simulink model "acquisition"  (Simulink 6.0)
settings: Solver=FixedStepDiscrete  StartTime=0  StopTime=80  FixedStep=Te  RelTol=1e-3
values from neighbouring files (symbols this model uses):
  Te = 0.1    [binome18.m]
undefined symbols (not defined in the file or in its folder): MIO, National_Instruments, PCI, sauvegarde_acquisition
libraries: simulink x6, rtwinlib x2, commseqgen2 x1

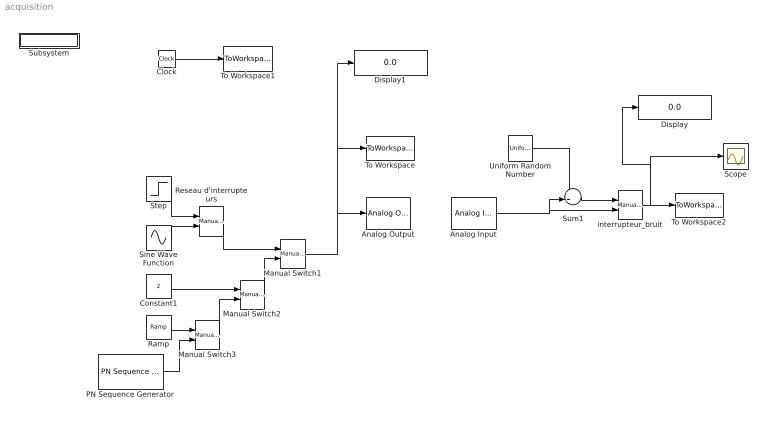
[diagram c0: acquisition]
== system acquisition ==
  Analog Input : rtwinlib/Analog Input  SampleTime=Te  DrvName=National_Instruments/PCI-MIO-16E-4  DrvAddress=4294967295  DrvOptions=[0 0 0]  Channels=1  RangeMode=1  VoltRange=1
  Analog Output : rtwinlib/Analog Output  SampleTime=Te  DrvName=National_Instruments/PCI-MIO-16E-4  DrvAddress=4294967295  DrvOptions=[0 0 0]  Channels=1  RangeMode=1  VoltRange=1  InitialValue=[]  FinalValue=0
  Clock : Clock
  Constant1 : Constant  Value=2
  Display : Display
  Display1 : Display
  Manual Switch1 : simulink/Signal Routing/Manual Switch  sw=1  action=0
  Manual Switch2 : simulink/Signal Routing/Manual Switch  sw=0  action=0
  Manual Switch3 : simulink/Signal Routing/Manual Switch  sw=1  action=0
  PN Sequence Generator : commseqgen2/PN Sequence Generator  poly=[1 0 0 0 0 1 1]  ini_sta=[0 0 0 0 0 1]  shift=0  Ts=Te  frameBased=off  sampPerFrame=1  reset=off
  Ramp : simulink/Sources/Ramp  slope=0.1  start=0  X0=0
  Reseau d'interrupteurs : simulink/Signal Routing/Manual Switch  sw=1  action=0
  Scope : Scope
  Sine Wave Function : Sin  Frequency=5  SampleTime=Te
  Step : Step  Time=5  Before=1  After=2  SampleTime=Te
  Subsystem : Subsystem  StopFcn=save sauvegarde_acquisition
  Sum1 : Sum  Inputs=++|
  To Workspace : ToWorkspace  VariableName=entreeVentilo  SampleTime=-1  SaveFormat=Array
  To Workspace1 : ToWorkspace  VariableName=t  SampleTime=Te  SaveFormat=Array
  To Workspace2 : ToWorkspace  VariableName=sortieVentilo  SampleTime=Te  SaveFormat=Array
  Uniform Random Number : UniformRandomNumber  Minimum=-0.4  Maximum=0.4  SampleTime=Te
  interrupteur_bruit : simulink/Signal Routing/Manual Switch  sw=0  action=0
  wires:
  Analog Input/1 -> interrupteur_bruit/2, Sum1/2
  Uniform Random Number/1 -> Sum1/1
  Sum1/1 -> interrupteur_bruit/1
  interrupteur_bruit/1 -> Display/1, Scope/1, To Workspace2/1
  Clock/1 -> To Workspace1/1
  Step/1 -> Reseau d'interrupteurs/1
  Sine Wave Function/1 -> Reseau d'interrupteurs/2
  Reseau d'interrupteurs/1 -> Manual Switch1/1
  Manual Switch1/1 -> Analog Output/1, To Workspace/1, Display1/1
  Manual Switch2/1 -> Manual Switch1/2
  Constant1/1 -> Manual Switch2/1
  Manual Switch3/1 -> Manual Switch2/2
  Ramp/1 -> Manual Switch3/1
  PN Sequence Generator/1 -> Manual Switch3/2

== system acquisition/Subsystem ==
